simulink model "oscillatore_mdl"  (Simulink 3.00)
settings: Solver=ode23s  StartTime=0.0  StopTime=10.0  RelTol=1e-6  AbsTol=1e-6
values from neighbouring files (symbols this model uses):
  beta = 60    [oscillatore.m]    (also in oscillatore_RC.m = 100; oscillatore_wien.m = 3.5)
  C = 0.001    [oscillatore.m]    (also in oscillatore_RC.m; oscillatore_RC_1.m; oscillatore_wien.m)
  Q30 = C*V30    (= 0.0001)    [oscillatore.m]    (also in oscillatore_RC.m; oscillatore_RC_1.m)
  R = 1    [oscillatore.m]    (also in oscillatore_RC.m; oscillatore_RC_1.m; oscillatore_wien.m)
  tau = 0.00001    (= 1e-05)    [oscillatore.m]    (also in oscillatore_RC.m)
  VM = 12    [oscillatore.m]    (also in oscillatore_RC.m; oscillatore_RC_1.m; oscillatore_wien.m)

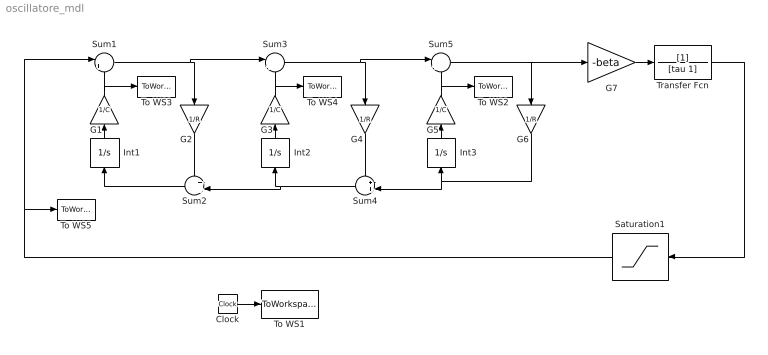
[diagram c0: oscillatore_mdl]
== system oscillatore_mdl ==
  Clock : Clock
  G1 : Gain  Orientation=up  Gain=1/C  SaturateOnIntegerOverflow=on
  G2 : Gain  Orientation=down  Gain=1/R  SaturateOnIntegerOverflow=on
  G3 : Gain  Orientation=up  Gain=1/C  SaturateOnIntegerOverflow=on
  G4 : Gain  Orientation=down  Gain=1/R  SaturateOnIntegerOverflow=on
  G5 : Gain  Orientation=up  Gain=1/C  SaturateOnIntegerOverflow=on
  G6 : Gain  Orientation=down  Gain=1/R  SaturateOnIntegerOverflow=on
  G7 : Gain  Gain=-beta  SaturateOnIntegerOverflow=on
  Int1 : Integrator  Orientation=up  ExternalReset=none  InitialConditionSource=internal  InitialCondition=0  LimitOutput=off  UpperSaturationLimit=inf  LowerSaturationLimit=-inf  ShowSaturationPort=off  ShowStatePort=off  AbsoluteTolerance=auto
  Int2 : Integrator  Orientation=up  ExternalReset=none  InitialConditionSource=internal  InitialCondition=0  LimitOutput=off  UpperSaturationLimit=inf  LowerSaturationLimit=-inf  ShowSaturationPort=off  ShowStatePort=off  AbsoluteTolerance=auto
  Int3 : Integrator  Orientation=up  ExternalReset=none  InitialConditionSource=internal  InitialCondition=Q30  LimitOutput=off  UpperSaturationLimit=inf  LowerSaturationLimit=-inf  ShowSaturationPort=off  ShowStatePort=off  AbsoluteTolerance=auto
  Saturation1 : Saturate  Orientation=left  UpperLimit=VM  LowerLimit=-VM
  Sum1 : Sum  Inputs=|+-  SaturateOnIntegerOverflow=on
  Sum2 : Sum  Orientation=left  Inputs=++|  SaturateOnIntegerOverflow=on
  Sum3 : Sum  Inputs=|+-  SaturateOnIntegerOverflow=on
  Sum4 : Sum  Orientation=left  Inputs=++|  SaturateOnIntegerOverflow=on
  Sum5 : Sum  Inputs=|+-  SaturateOnIntegerOverflow=on
  To WS1 : ToWorkspace  VariableName=t  SampleTime=-1  SaveFormat=Matrix
  To WS2 : ToWorkspace  VariableName=V3  SampleTime=-1  SaveFormat=Matrix
  To WS3 : ToWorkspace  VariableName=V1  SampleTime=-1  SaveFormat=Matrix
  To WS4 : ToWorkspace  VariableName=V2  SampleTime=-1  SaveFormat=Matrix
  To WS5 : ToWorkspace  VariableName=Vp  SampleTime=-1  SaveFormat=Matrix
  Transfer Fcn : TransferFcn  Numerator=[1]  Denominator=[tau 1]
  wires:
  Int1/1 -> G1/1
  G2/1 -> Sum2/1
  Sum2/1 -> Int1/1
  Sum1/1 -> G2/1, Sum3/1
  Int2/1 -> G3/1
  G4/1 -> Sum4/1
  Sum3/1 -> G4/1, Sum5/1
  Int3/1 -> G5/1
  Sum4/1 -> Int2/1, Sum2/2
  G6/1 -> Int3/1, Sum4/2
  Sum5/1 -> G6/1, G7/1
  G7/1 -> Transfer Fcn/1
  Clock/1 -> To WS1/1
  G1/1 -> Sum1/2, To WS3/1
  G3/1 -> Sum3/2, To WS4/1
  G5/1 -> Sum5/2, To WS2/1
  Transfer Fcn/1 -> Saturation1/1
  Saturation1/1 -> Sum1/1, To WS5/1
